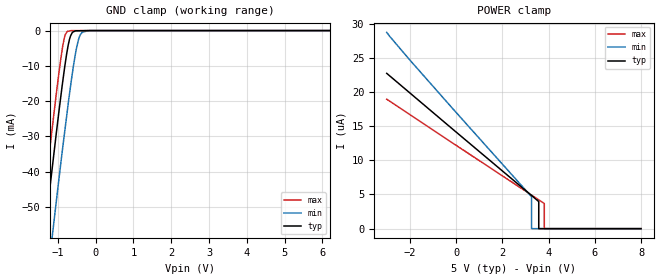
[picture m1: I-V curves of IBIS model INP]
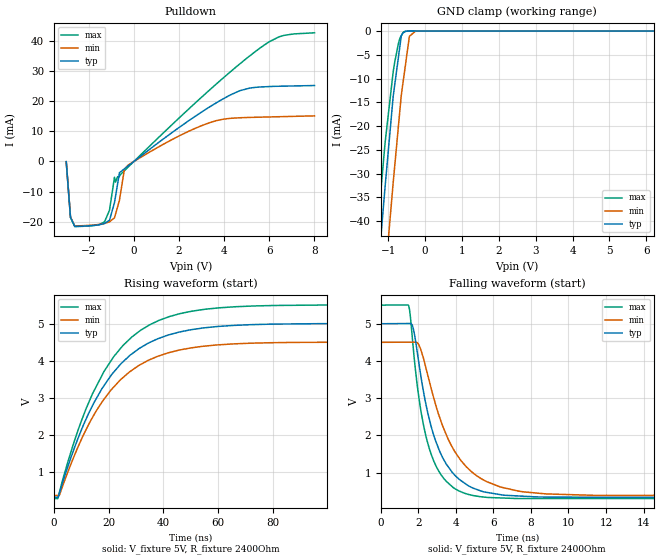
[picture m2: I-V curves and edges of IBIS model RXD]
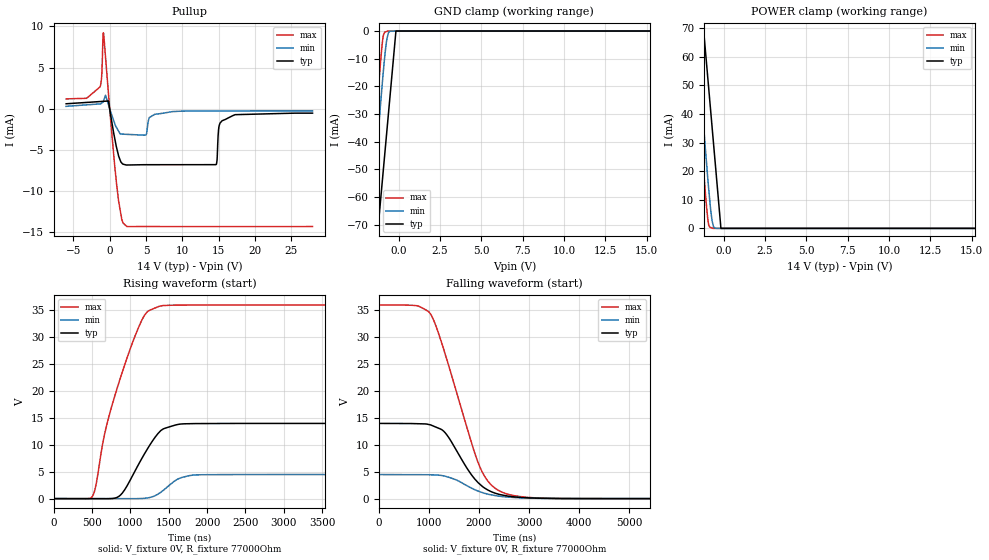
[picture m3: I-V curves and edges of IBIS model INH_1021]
|Texas Instruments Incorporated
|TLIN1021-Q1 Local Interconnect Network (LIN) Transceiver with Dominant
|State Timeout
[IBIS Ver]   4.1
[File name]   tlin1021-q1.ibs
[Date]   12/12/2019
[File Rev]   1.0
[Source]
| Texas Instruments Incorporated.
| Analog-eLab Design Center, HPA
| 12500 TI Blvd
| Dallas, TX -75243
[Notes]
| Rev 1.0: 12/12/2019
| - Initial version of the model
| - Model generated from simulations in SPECTRE
| - Model matched to SPICE simulation
| - C_comp although listed in numerical order of value are
|   obtained from varying PVT conditions. For PVT conditions for
|   each specific value refer the buffer description under
|   respective [Model]. IBIS model user is responsible for using
|   appropriate C_comp to simulate for Signal Integrity.
| - Warnings regarding combined Non-monotonicity of various models
|   have been reviewed and considered minor and can be ignored.
| - LIN_OD Models should be used when there is an external pullup present on the LIN Bus.
| - LIN_CMOS models should be used when there is no external pullup present on the LIN Bus.
[Disclaimer]
| This model is designed as an aid for customers of Texas Instruments.
| TI and its licensors and suppliers make no warranties, either expressed
| or implied, with respect to this  model, including the warranties of
| merchantability or fitness for a particular purpose. The model is
| provided solely on an "as is" basis. The entire risk as to its quality
| and performance is with the customer.
[Copyright]
(C) Copyright 2019 Texas Instruments Incorporated.All rights reserved.
|  Component TLIN1021DRQ1 8-pin SOIC - D package
|  Part # TLIN1021DRQ1
[Component]   TLIN1021DRQ1
[Manufacturer]  TI
[Package]   |8 SOIC - D package
|   typ   min   max
R_pkg   0.1   0.08   0.12
L_pkg   1.0nH   0.8nH   1.2nH
C_pkg   0.2pF   0.16pF   0.24pF
[Pin]  signal_name model_name   R_pin   L_pin   C_pin
1   RXD   RXD   NA   NA   NA
2   EN   INP   NA   NA   NA
3   WAKE   WAKE   NA   NA   NA
4   TXD   INP   NA   NA   NA
5   GND   gnd   NA   NA   NA
6   LIN   LIN   NA   NA   NA
7   VSUP   power   NA   NA   NA
8   INH   INH   NA   NA   NA
|  Component TLIN1021DRBRQ1 8-pin VSON - DRB package
|  Part # TLIN1021DRBRQ1
[Component]   TLIN1021DRBRQ1
[Manufacturer]  TI
[Package]   |8 VSON - DRB package
|   typ   min   max
R_pkg   0.1   0.08   0.12
L_pkg   1.0nH   0.8nH   1.2nH
C_pkg   0.2pF   0.16pF   0.24pF
[Pin]  signal_name model_name   R_pin   L_pin   C_pin
1   RXD   RXD   NA   NA   NA
2   EN   INP   NA   NA   NA
3   WAKE   WAKE   NA   NA   NA
4   TXD   INP   NA   NA   NA
5   GND   gnd   NA   NA   NA
6   LIN   LIN   NA   NA   NA
7   VSUP   power   NA   NA   NA
8   INH   INH   NA   NA   NA
|   Model Selectors
[Model Selector] INH
INH_1021   14.0V   1021 Range
INH_14p0   14.0V   Nominal 14V VSUP
[Model Selector] WAKE
WAKE_1021   14.0V   1021 Range
WAKE_14p0   14.0V   Nominal 14V VSUP
[Model Selector] LIN
LIN_CMOS   14.0V   1021 Range
LIN_CMOS_14p0   14.0V   Nominal 14V VSUP
LIN_OD   14.0V   1021 Range
LIN_OD_14p0   14.0V   Nominal 14V VSUP
| Models and submodels in the file (10): INP (Input), RXD (Open_sink), INH_1021 (Open_source), INH_14p0 (Open_source), WAKE_1021 (Input), WAKE_14p0 (Input), LIN_OD (I/O_open_drain), LIN_OD_14p0 (I/O_open_drain), LIN_CMOS (Output), LIN_CMOS_14p0 (Output)
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|   INP
[Model]   INP
Model_type   Input
Vinl = 0.8
Vinh = 2
|   typ   min   max
C_comp   3.46465E-12  3.07372E-12  4.01486E-12
[Voltage Range]   5   4.5   5.5
[Temperature Range]   25   165   -55
[Power Clamp Reference]   5   4.5   5.5
[GND Clamp Reference]   0   0   0
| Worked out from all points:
|   GND clamp passes 1 mA (typ) near -0.64 V on its own axis
[GND Clamp]
|   Voltage   I(typ)   I(min)   I(max)
-3V       -217.2mA   -236mA     -206.6mA
-1.51V    -72.76mA   -92.22mA   -61.59mA
-1.445V   -66.59mA   -86mA      -55.38mA
-1.318V   -54.67mA   -74.08mA   -43.45mA
-1.118V   -36.14mA   -55.55mA   -24.84mA
-866.8mV  -14.16mA   -32.81mA   -4.138mA
-739.2mV  -4.935mA   -21.91mA   -208.8uA
-665.4mV  -1.562mA   -15.88mA   -38.48uA
-510.7mV  -66.04uA   -5.215mA   -13.79uA
-432.9mV  -50.97uA   -1.899mA   -10.94uA
-346.1mV  -34.13uA   -380.5uA   -7.754uA
8V        0A         0A         0A
[POWER Clamp]
|   Voltage   I(typ)   I(min)   I(max)
-3V       22.73uA    28.72uA    18.94uA
3.262V    4.861uA    4.674uA    4.917uA
3.264V    4.856uA    4.553uA    4.912uA
3.264V    4.856uA    1.308uA    4.912uA
3.265V    4.853uA    0A         4.91uA
3.574V    3.965uA    0A         4.22uA
3.575V    3.714uA    0A         4.219uA
3.575V    0A         0A         4.218uA
3.815V    0A         0A         3.677uA
3.816V    0A         0A         3.566uA
3.816V    0A         0A         0A
8V        0A         0A         0A
|   RXD Model
[Model]   RXD
Model_type   Open_sink
Polarity   Non-Inverting
Vmeas = 2.5
Vref = 5
Cref = 0pF
Rref = 2400
|   typ   min   max
C_comp   3.72956E-12  3.27827E-12  4.2623E-12
[Voltage Range]   5   4.5   5.5
[Temperature Range]   25   165   -55
[Pullup Reference]   5   4.5   5.5
[Pulldown Reference]   0   0   0
[Power Clamp Reference]   5   4.5   5.5
[GND Clamp Reference]   0   0   0
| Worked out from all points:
|   slope of the pulldown table from 0 to 0.75 V, typ, clamps not added: 173 ohm
|   GND clamp passes 1 mA (typ) near -0.64 V on its own axis
|   falling waveform, V_fixture 5V, R_fixture 2400Ohm: 20-80 % time 1.45ns typ, 2ns min, 1.09ns max; typ from 5 V to 0.333 V
|   rising waveform, V_fixture 5V, R_fixture 2400Ohm: 20-80 % time 21ns typ, 21.1ns min, 20.6ns max; typ from 0.333 V to 5 V
[Pulldown]
|   Voltage   I(typ)   I(min)   I(max)
-3V       -91.95uA   -51.84uA   -125.3uA
-2.811V   -18.55mA   -18.44mA   -18.62mA
-2.622V   -21.54mA   -21.41mA   -21.62mA
-1.522V   -21mA      -20.89mA   -20.91mA
-1.082V   -19.51mA   -20.05mA   -16.18mA
-862mV    -13.66mA   -18.71mA   -5.223mA
-642mV    -3.734mA   -12.89mA   -4.892mA
-422mV    -2.458mA   -2.58mA    -3.081mA
-253.3mV  -1.479mA   -1.17mA    -1.849mA
1.886V    10.65mA    8.023mA    13.61mA
5.997V    24.84mA    14.76mA    39.72mA
8V        25.19mA    15.12mA    42.68mA
[GND Clamp]
|   Voltage   I(typ)   I(min)   I(max)
-3V       -217.2mA   -235.8mA   -207mA
-1.302V   -53.19mA   -72.29mA   -43.06mA
-1.082V   -32.87mA   -51.83mA   -23.57mA
-862mV    -13.78mA   -31.95mA   -8.605mA
-815.1mV  -11.06mA   -28.01mA   -6.361mA
-721.3mV  -5.616mA   -20.15mA   -2.686mA
-674.4mV  -2.896mA   -16.21mA   -1.392mA
-642mV    -1.017mA   -13.49mA   -976.1uA
-580.6mV  -322.1uA   -10.04mA   -187.4uA
-422mV    -9uA       -1.107mA   -3.295uA
-253.3mV  53.27nA    -15.43uA   76.49nA
8V        58.21nA    81.53nA    58.68nA
[Ramp]
R_load = 2400
|   typ   min   max
dV/dt_r   2.80006/2.10383e-08   2.47249/2.11506e-08   3.12257/2.06129e-08
dV/dt_f   2.80006/1.44933e-09   2.47249/1.99612e-09   3.12257/1.09155e-09
[Falling Waveform]
V_fixture = 5V
V_fixture_min = 4.5V
V_fixture_max = 5.5V
R_fixture = 2400Ohm
C_fixture = 0F
|   Time   V(typ)   V(min)   V(max)
0s        5V         4.5V       5.5V
1.491ns   5.005V     4.504V     5.484V
1.724ns   4.895V     4.505V     4.401V
2.078ns   3.795V     4.378V     2.862V
2.697ns   2.22V      3.242V     1.478V
3.655ns   1.113V     1.832V     689.4mV
4.933ns   577.8mV    982.7mV    380.1mV
7.334ns   369.1mV    500.1mV    299.6mV
11.34ns   334.5mV    386.2mV    299.6mV
50ns      333.2mV    379.1mV    295.7mV
[Rising Waveform]
V_fixture = 5V
V_fixture_min = 4.5V
V_fixture_max = 5.5V
R_fixture = 2400Ohm
C_fixture = 0F
|   Time   V(typ)   V(min)   V(max)
0s        333.2mV    379.1mV    295.7mV
1.397ns   331mV      378.1mV    292mV
2.057ns   440.2mV    389.4mV    467.2mV
6.668ns   1.482V     1.298V     1.646V
11.68ns   2.414V     2.134V     2.69V
21.93ns   3.697V     3.295V     4.113V
34.94ns   4.487V     4.024V     4.961V
55.34ns   4.887V     4.394V     5.384V
100.4ns   4.997V     4.496V     5.498V
600ns     5V         4.5V       5.5V
|   INH_1021
[Model]   INH_1021
Model_type   Open_source
Polarity   Non-Inverting
Vmeas = 2.5
Vref = 2.5
Cref = 2pF
Rref = 77000
|   typ   min   max
C_comp   1.675pF   1.271pF   2.536pF
[Voltage Range]   14   4.5   36
[Temperature Range]   25   165   -55
[Pullup Reference]   14   4.5   36
[Pulldown Reference]   0   0   0
[Power Clamp Reference]   14   4.5   36
[GND Clamp Reference]   0   0   0
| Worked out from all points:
|   slope of the pullup table from 0 to 2.1 V, typ, clamps not added: 309 ohm
|   GND clamp passes 1 mA (typ) near -0.18 V on its own axis
|   POWER clamp passes 1 mA (typ) near -0.18 V on its own axis
|   falling waveform, V_fixture 0V, R_fixture 77000Ohm: 20-80 % time 596ns typ, 639ns min, 703ns max; typ from 14 V to 0 V
|   rising waveform, V_fixture 0V, R_fixture 77000Ohm: 20-80 % time 338ns typ, 247ns min, 419ns max; typ from 0 V to 14 V
[GND Clamp]
|   Voltage   I(typ)   I(min)   I(max)
-6V       -446mA     -447.3mA   -446.1mA
-1.885V   -113.4mA   -87.75mA   -73.56mA
-1.713V   -102mA     -74.04mA   -59.49mA
-1.446V   -84.46mA   -53.12mA   -38.07mA
-1.239V   -70.79mA   -37.12mA   -22.01mA
-1.079V   -60.21mA   -25.28mA   -10.03mA
-950.6mV  -51.78mA   -16.22mA   -2.45mA
-787.6mV  -41.04mA   -6.241mA   -284.1uA
-650.5mV  -32.01mA   -1.386mA   -9.232uA
-567.8mV  -26.55mA   -239.8uA   -8.135uA
-164.9mV  0A         -14.26uA   -2.793uA
36V       0A         0A         0A
[Pullup]
|   Voltage   I(typ)   I(min)   I(max)
-6V       616.7uA    305.1uA    1.21mA
-1.349V   886.3uA    603.3uA    2.65mA
-1.124V   899.3uA    683.7uA    3.667mA
-864.8mV  914.4uA    930.9uA    9.231mA
-164.9mV  954.9uA    486.3uA    1.817mA
1.22V     -5.676mA   -2.694mA   -11.12mA
2.391V    -6.817mA   -3.096mA   -14.29mA
6.211V    -6.779mA   -662.3uA   -14.29mA
14.65V    -6.765mA   -252.3uA   -14.29mA
15.05V    -2.237mA   -251.7uA   -14.29mA
15.5V     -1.44mA    -251uA     -14.29mA
27.96V    -518.4uA   -243.2uA   -14.29mA
[POWER Clamp]
|   Voltage   I(typ)   I(min)   I(max)
-6V       447.1mA    448.6mA    447mA
-1.885V   113.8mA    88.82mA    74.36mA
-1.713V   102.4mA    75.03mA    60.23mA
-1.446V   84.79mA    53.96mA    38.68mA
-1.239V   71.07mA    37.85mA    22.52mA
-1.129V   63.79mA    29.56mA    14.11mA
-1.029V   57.14mA    22.32mA    7.117mA
-930.8mV  50.67mA    15.45mA    2.005mA
-762.1mV  39.52mA    5.378mA    267.8uA
-650.5mV  32.13mA    1.46mA     14.74uA
-164.9mV  0A         6.081uA    4.459uA
36V       0A         0A         0A
[Ramp]
R_load = 77000
|   typ   min   max
dV/dt_r   8.38087/3.3827e-07   2.68785/2.47073e-07   21.5739/4.18892e-07
dV/dt_f   8.38087/5.96252e-07   2.68785/6.3461e-07   21.5739/7.02977e-07
[Falling Waveform]
V_fixture = 0V
V_fixture_min = 0V
V_fixture_max = 0V
R_fixture = 77000Ohm
C_fixture = 0F
|   Time   V(typ)   V(min)   V(max)
0s        13.97V     4.48V      35.96V
753.9ns   13.92V     4.455V     35.82V
1.028us   13.71V     4.438V     34.34V
1.322us   12.26V     4.17V      26.9V
1.784us   5.311V     2.285V     12.42V
2.018us   2.676V     1.279V     5.872V
2.226us   1.385V     742mV      2.728V
2.49us    638.9mV    368.4mV    1.1V
3.518us   42.89mV    41.01mV    53.71mV
9.9us     7.126uV    30.62uV    26.91uV
[Rising Waveform]
V_fixture = 0V
V_fixture_min = 0V
V_fixture_max = 0V
R_fixture = 77000Ohm
C_fixture = 0F
|   Time   V(typ)   V(min)   V(max)
0s        8.018uV    29.75uV    26.3uV
509ns     -8.413mV   -3.507mV   565.3mV
696.5ns   -11.23mV   -4.81mV    14.04V
867.5ns   632.3mV    -5.998mV   22.36V
998.2ns   3.489V     -6.907mV   27.86V
1.181us   8.285V     57.47mV    34.03V
1.389us   12.54V     1.118V     35.75V
1.622us   13.77V     3.662V     35.91V
1.898us   13.93V     4.423V     35.94V
9.9us     13.97V     4.48V      35.96V
